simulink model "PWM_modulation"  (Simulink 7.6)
settings: Solver=ode45  StartTime=0.0  StopTime=0.02  RelTol=1e-3
libraries: fl_lib x5, nesl_utility x4, elec_lib x1, simulink x1

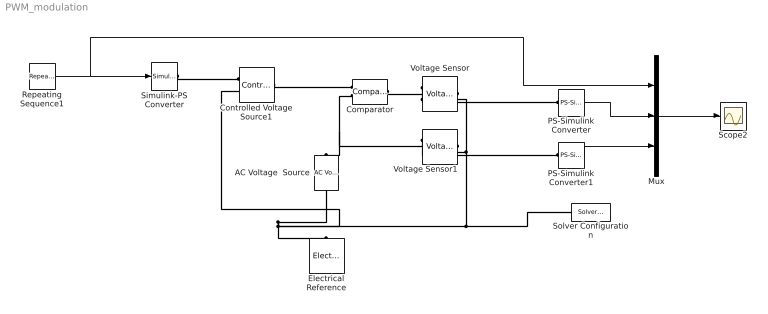
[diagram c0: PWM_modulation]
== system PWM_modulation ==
  AC Voltage  Source : fl_lib/Electrical/Electrical Sources/AC Voltage Source  DialogController=NetworkEngine.DynNeDlgSource  SystemSampleTime=-1  amp=1 V  shift=0 rad  omega=120 Hz  i_Log=off  v_Log=off  LocalVarNames=|i|v  LocalVarDescs=|i|v  LocalVarLogging=[0 0]
  Comparator : elec_lib/Integrated Circuits/Comparator  DialogController=NetworkEngine.DynNeDlgSource  SystemSampleTime=-1  V_OS=5 mV  V_OL=0 V  V_OH=5 V  C_IN=0 pF  R_OUT=50 Ohm  Delay=0 s  LocalVarLogging=[]
  Controlled Voltage Source1 : fl_lib/Electrical/Electrical Sources/Controlled Voltage Source  DialogController=NetworkEngine.DynNeDlgSource  SystemSampleTime=-1  i_Log=off  v_Log=off  LocalVarNames=|i|v  LocalVarDescs=|i|v  LocalVarLogging=[0 0]
  Electrical Reference : fl_lib/Electrical/Electrical Elements/Electrical Reference  DialogController=NetworkEngine.DynNeDlgSource  SystemSampleTime=-1  i_Log=off  LocalVarNames=|i  LocalVarDescs=|i  LocalVarLogging=0
  Mux : Mux  Inputs=3
  PS-Simulink Converter : nesl_utility/PS-Simulink Converter  DialogController=NetworkEngine.DynNeUtilDlgSource  SystemSampleTime=-1  PhysicalDomain=network_engine_domain  LeftPortType=input  RightPortType=output  SubClassName=ps_output  Unit=1  AffineConversion=off
  PS-Simulink Converter1 : nesl_utility/PS-Simulink Converter  DialogController=NetworkEngine.DynNeUtilDlgSource  SystemSampleTime=-1  PhysicalDomain=network_engine_domain  LeftPortType=input  RightPortType=output  SubClassName=ps_output  Unit=1  AffineConversion=off
  Repeating Sequence1 : simulink/Sources/Repeating Sequence  SystemSampleTime=-1  rep_seq_t=[0 0.001]  rep_seq_y=[0 1]
  Scope2 : Scope
  Simulink-PS Converter : nesl_utility/Simulink-PS Converter  DialogController=NetworkEngine.DynNeUtilDlgSource  SystemSampleTime=-1  PhysicalDomain=network_engine_domain  LeftPortType=input  RightPortType=output  SubClassName=ps_input  Unit=1  AffineConversion=off  InputFilterTimeConstant=.001  UdotUserProvided=0
  Solver Configuration : nesl_utility/Solver Configuration  DialogController=NetworkEngine.DynNeUtilDlgSource  SystemSampleTime=-1  PhysicalDomain=network_engine_domain  LeftPortType=input  RightPortType=generic  SubClassName=solver  Accelerate=off  Profile=off  ResidualTolerance=1e-9  MaxNonlinIter=12  MaxModeIter=2  DoFixedCost=off  UseLocalSampling=off  DoDC=off  LinearAlgebra=Sparse  LocalSolverSampleTime=.001  LocalSolverChoice=NE_BACKWARD_EULER_ADVANCER  UseLocalSolver=off
  Voltage Sensor : fl_lib/Electrical/Electrical Sensors/Voltage Sensor  DialogController=NetworkEngine.DynNeDlgSource  SystemSampleTime=-1  i1_Log=off  v1_Log=off  LocalVarNames=|i1|v1  LocalVarDescs=|i1|v1  LocalVarLogging=[0 0]
  Voltage Sensor1 : fl_lib/Electrical/Electrical Sensors/Voltage Sensor  DialogController=NetworkEngine.DynNeDlgSource  SystemSampleTime=-1  i1_Log=off  v1_Log=off  LocalVarNames=|i1|v1  LocalVarDescs=|i1|v1  LocalVarLogging=[0 0]
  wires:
  Repeating Sequence1/1 -> Simulink-PS Converter/1, Mux/1
  Mux/1 -> Scope2/1
  PS-Simulink Converter1/1 -> Mux/3
  PS-Simulink Converter/1 -> Mux/2
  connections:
  Simulink-PS Converter/RConn1 -- Controlled Voltage Source1/RConn1
  Controlled Voltage Source1/LConn1 -- Comparator/LConn1
  Comparator/LConn2 -- AC Voltage  Source/LConn1 -- Voltage Sensor1/LConn1
  Voltage Sensor/RConn2 -- Solver Configuration/RConn1 -- AC Voltage  Source/RConn1 -- Electrical Reference/LConn1 -- Controlled Voltage Source1/RConn2 -- Voltage Sensor1/RConn2
  Comparator/RConn1 -- Voltage Sensor/LConn1
  Voltage Sensor/RConn1 -- PS-Simulink Converter/LConn1
  Voltage Sensor1/RConn1 -- PS-Simulink Converter1/LConn1
